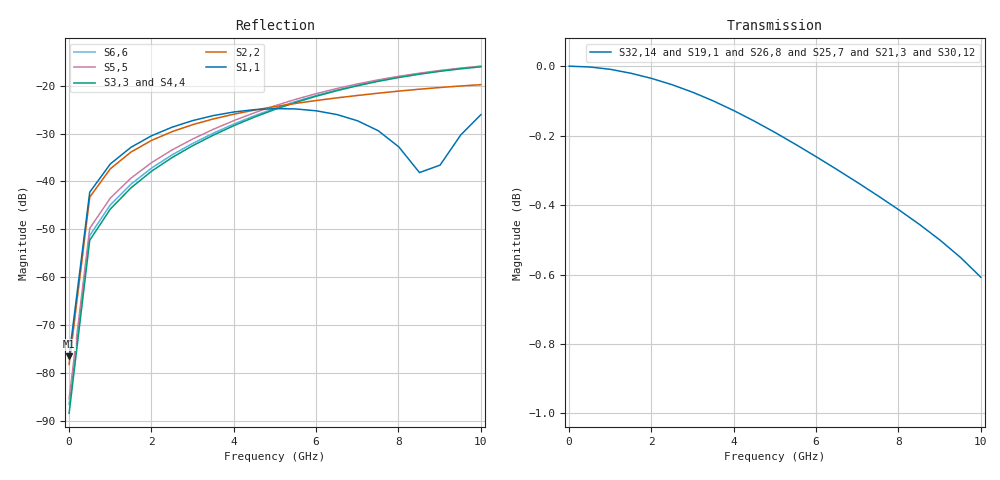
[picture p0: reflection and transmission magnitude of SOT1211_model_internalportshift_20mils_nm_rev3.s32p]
! Touchstone file from project SOT1211_model_internalportshift_20mils_rev3
! Exported from HFSS 15.0.0
! Variables:
!  Gate_Lead_Shift = 1000um
!  PCB_H = 760um
!  PCB_Metal_H = 100um
# GHZ S MA R 50.000000
! Terminal data exported
! Port[1] = Box3_T1
! Port[2] = Box4_T1
! Port[3] = Box5_T1
! Port[4] = Box6_T1
! Port[5] = Box7_T1
! Port[6] = Box8_T1
! Port[7] = Box9_T1
! Port[8] = Box10_T1
! Port[9] = Box11_T1
! Port[10] = Box12_T1
! Port[11] = Box13_T1
! Port[12] = Box14_T1
! Port[13] = Box15_T1
! Port[14] = Box16_T1
! Port[15] = Box19_T1
! Port[16] = Box20_T1
! Port[17] = Rectangle1_T1
! Port[18] = Rectangle2_T1
! Port[19] = Rectangle3_T1
! Port[20] = Rectangle4_T1
! Port[21] = Rectangle5_T1
! Port[22] = Rectangle6_T1
! Port[23] = Rectangle7_T1
! Port[24] = Rectangle8_T1
! Port[25] = Rectangle9_T1
! Port[26] = Rectangle10_T1
! Port[27] = Rectangle11_T1
! Port[28] = Rectangle12_T1
! Port[29] = Rectangle13_T1
! Port[30] = Rectangle14_T1
! Port[31] = Rectangle15_T1
! Port[32] = Rectangle16_T1
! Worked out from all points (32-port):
!   21 points, 10 MHz to 10 GHz, reference 50 ohm
!   strongest paths, dB at 10 MHz, 2.51 GHz, 5.01 GHz, 7.51 GHz, 10 GHz:
!     S32,14: 0.0, -0.1, -0.2, -0.4, -0.6
!     S19,1: 0.0, -0.1, -0.2, -0.4, -0.6
!     S26,8: 0.0, -0.1, -0.2, -0.4, -0.6
!     S25,7: 0.0, -0.1, -0.2, -0.4, -0.6
!     S21,3: 0.0, -0.1, -0.3, -0.5, -0.8
!     S30,12: 0.0, -0.1, -0.3, -0.5, -0.8
!   lowest |S11| = -76.6 dB at 10 MHz (marker M1), VSWR 1.00, Z = 50 - j0.0146 ohm
!   |S11| at or under -10 dB: start of sweep to end of sweep
